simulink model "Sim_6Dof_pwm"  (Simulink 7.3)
settings: Solver=ode4  StartTime=0.0  StopTime=80  FixedStep=0.0005  MaxStep=0.0005  RelTol=1e-3
InitFcn:
  | run
StartFcn:
  | run
StopFcn:
  | Pl
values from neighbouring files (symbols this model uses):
  calfa = cos(alfa0*d2r)    [run.m]
  d2r = pi/180    (= 0.0174532925199)    [run.m]
  Kfilt = (wd1^2*wd2^2*wd3^2*wd4^2*wd5^2*wd6^2)/(wn1^2*wn2^2*wn3^2*wn4^2*wn5^2*wn6^2)    (= 0.818930549142)    [run.m]
  klr = lqr(Ap4,Bp4,Q,R)    [run.m]
  kls = lqr(Ap3,Bp3,Q,R)    [run.m]
  r2d = 180/pi    (= 57.2957795131)    [Pl.m]    (also in run.m)
  salfa = sin(alfa0*d2r)    [run.m]
  Thet0 = 43    [run.m]
  V0 = 18640    [run.m]
  wd1 = 29    [run.m]
  wd2 = 37    [run.m]
  wd3 = 40    [run.m]
  wd4 = 48    [run.m]
  wd5 = 63    [run.m]
  wd6 = 68    [run.m]
  wd7 = 34    [run.m]
  wd8 = 19.1    [run.m]
  wlp = 6.6    [run.m]
  wlp2 = 12    [run.m]
  wlpr = 12    [run.m]
  wn1 = 30    [run.m]
  wn2 = 37.9    [run.m]
  wn3 = 40.2    [run.m]
  wn4 = 48.6    [run.m]
  wn5 = 64    [run.m]
  wn6 = 68.6    [run.m]
  wn7 = 34    [run.m]
  wn8 = 19.1    [run.m]
  zd1 = 0.12    [run.m]
  zd2 = 0.12    [run.m]
  zd3 = 0.1    [run.m]
  zd4 = 0.1    [run.m]
  zd5 = 0.1    [run.m]
  zd6 = 0.1    [run.m]
  zd7 = 0.1    [run.m]
  zd8 = 0.1    [run.m]
  zlp = 0.9    [run.m]
  zlp2 = 0.7    [run.m]
  zlpr = 0.7    [run.m]
  zn1 = 0.008    [run.m]
  zn2 = 0.01    [run.m]
  zn3 = 0.01    [run.m]
  zn4 = 0.02    [run.m]
  zn5 = 0.01    [run.m]
  zn6 = 0.01    [run.m]
  zn7 = 0.01    [run.m]
  zn8 = 0.01    [run.m]
undefined symbols (not defined in the file or in its folder): Aai, Aao, Af, Bai, Bao, Bf, Cai, Cao, Cf, Dai, Dao, Df, KSmix, Pos_Thrust3
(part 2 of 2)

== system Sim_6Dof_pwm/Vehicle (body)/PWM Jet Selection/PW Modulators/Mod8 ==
  In1 : Inport  OutDataType=sfix(16)  OutScaling=2^0
  " " : Product  OutDataType=sfix(16)  OutScaling=2^0
  "  " : TransferFcn  Numerator=[5]  Denominator=[1/5 1]
  "   " : Constant  Value=1.001  OutDataType=sfix(16)  OutScaling=2^0
  "    " : Product  OutDataType=sfix(16)  OutScaling=2^0
  "    1" : Product  OutDataType=sfix(16)  OutScaling=2^0
  "   1" : Constant  Value=1.001  OutDataType=sfix(16)  OutScaling=2^0
  "  1" : TransferFcn  Numerator=[5]  Denominator=[1/5 1]
  " 1" : Product  OutDataType=sfix(16)  OutScaling=2^0
  0.5 : Gain  Gain=0.5  ParameterDataType=sfix(16)  ParameterScaling=2^0  OutDataType=sfix(16)  OutScaling=2^0
  Abs : Abs
  Abs1 : Abs
  Demux2 : Demux  Outputs=2
  Mem : Memory
  Mem1 : Memory
  Relay : Relay  OnSwitchValue=0.5  OffSwitchValue=0.5  OutDataType=sfix(16)  OutScaling=2^0
  Relay1 : Relay  OnSwitchValue=0.5  OffSwitchValue=0.5  OutDataType=sfix(16)  OutScaling=2^0
  Sign : Signum
  Sign1 : Signum
  Sum : Sum  Inputs=|+-  OutDataType=sfix(16)  OutScaling=2^0
  Sum1 : Sum  Inputs=|+-  OutDataType=sfix(16)  OutScaling=2^0
  Sum3 : Sum  Inputs=++|  OutDataType=sfix(16)  OutScaling=2^0
  O1 : Outport  OutDataType=sfix(16)  OutScaling=2^0
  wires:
  0.5/1 -> O1/1
  Sum3/1 -> 0.5/1
  In1/1 -> Demux2/1
  Demux2/1 -> " "/1
  Demux2/2 -> " 1"/1
  " 1"/1 -> Sum1/1
  "   1"/1 -> " 1"/2
  Sum1/1 -> "  1"/1
  "  1"/1 -> Abs1/1, Sign1/1
  Abs1/1 -> Relay1/1
  Relay1/1 -> "    1"/1
  Sign1/1 -> "    1"/2
  Mem1/1 -> Sum1/2
  "    1"/1 -> Sum3/2, Mem1/1
  " "/1 -> Sum/1
  "   "/1 -> " "/2
  Sum/1 -> "  "/1
  "  "/1 -> Abs/1, Sign/1
  Abs/1 -> Relay/1
  Relay/1 -> "    "/1
  Sign/1 -> "    "/2
  Mem/1 -> Sum/2
  "    "/1 -> Sum3/1, Mem/1

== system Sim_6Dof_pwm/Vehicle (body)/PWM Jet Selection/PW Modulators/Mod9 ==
  In1 : Inport  OutDataType=sfix(16)  OutScaling=2^0
  " " : Product  OutDataType=sfix(16)  OutScaling=2^0
  "  " : TransferFcn  Numerator=[5]  Denominator=[1/5 1]
  "   " : Constant  Value=1.001  OutDataType=sfix(16)  OutScaling=2^0
  "    " : Product  OutDataType=sfix(16)  OutScaling=2^0
  "    1" : Product  OutDataType=sfix(16)  OutScaling=2^0
  "   1" : Constant  Value=1.001  OutDataType=sfix(16)  OutScaling=2^0
  "  1" : TransferFcn  Numerator=[5]  Denominator=[1/5 1]
  " 1" : Product  OutDataType=sfix(16)  OutScaling=2^0
  0.5 : Gain  Gain=0.5  ParameterDataType=sfix(16)  ParameterScaling=2^0  OutDataType=sfix(16)  OutScaling=2^0
  Abs : Abs
  Abs1 : Abs
  Demux2 : Demux  Outputs=2
  Mem : Memory
  Mem1 : Memory
  Relay : Relay  OnSwitchValue=0.5  OffSwitchValue=0.5  OutDataType=sfix(16)  OutScaling=2^0
  Relay1 : Relay  OnSwitchValue=0.5  OffSwitchValue=0.5  OutDataType=sfix(16)  OutScaling=2^0
  Sign : Signum
  Sign1 : Signum
  Sum : Sum  Inputs=|+-  OutDataType=sfix(16)  OutScaling=2^0
  Sum1 : Sum  Inputs=|+-  OutDataType=sfix(16)  OutScaling=2^0
  Sum3 : Sum  Inputs=++|  OutDataType=sfix(16)  OutScaling=2^0
  O1 : Outport  OutDataType=sfix(16)  OutScaling=2^0
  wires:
  0.5/1 -> O1/1
  Sum3/1 -> 0.5/1
  In1/1 -> Demux2/1
  Demux2/1 -> " "/1
  Demux2/2 -> " 1"/1
  " 1"/1 -> Sum1/1
  "   1"/1 -> " 1"/2
  Sum1/1 -> "  1"/1
  "  1"/1 -> Abs1/1, Sign1/1
  Abs1/1 -> Relay1/1
  Relay1/1 -> "    1"/1
  Sign1/1 -> "    1"/2
  Mem1/1 -> Sum1/2
  "    1"/1 -> Sum3/2, Mem1/1
  " "/1 -> Sum/1
  "   "/1 -> " "/2
  Sum/1 -> "  "/1
  "  "/1 -> Abs/1, Sign/1
  Abs/1 -> Relay/1
  Relay/1 -> "    "/1
  Sign/1 -> "    "/2
  Mem/1 -> Sum/2
  "    "/1 -> Sum3/1, Mem/1
